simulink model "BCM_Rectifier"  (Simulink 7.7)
settings: Solver=ode45  StartTime=0.0  StopTime=5  RelTol=3e-14
libraries: fl_lib x5, nesl_utility x4, Memristor_lib x1

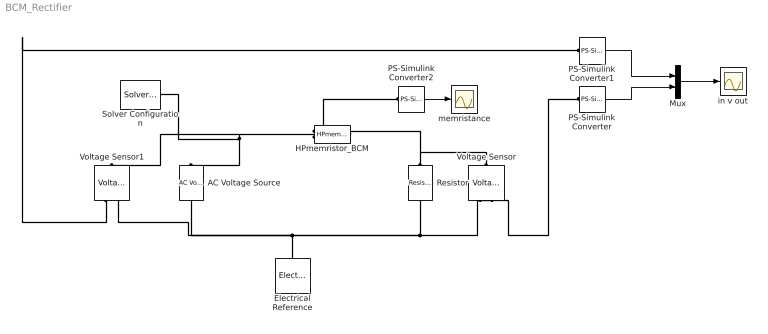
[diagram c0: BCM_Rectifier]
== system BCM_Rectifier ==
  AC Voltage Source : fl_lib/Electrical/Electrical Sources/AC Voltage Source  SystemSampleTime=-1  amp=1 V  shift=0 rad  omega=1 Hz  i_Log=off  v_Log=off  LocalVarNames=|i|v  LocalVarDescs=|i|v  LocalVarLogging=[0 0]
  Electrical Reference : fl_lib/Electrical/Electrical Elements/Electrical Reference  SystemSampleTime=-1  i_Log=off  LocalVarNames=|i  LocalVarDescs=|i  LocalVarLogging=0
  HPmemristor_BCM : Memristor_lib/HPmemristor_BCM  SystemSampleTime=-1  G_off=6e-5 1/Ohm  G_on=0.5 1/Ohm  N=1 1/Ohm  u_v=1e-10 m^2/s/V  D=1e-8 m  x0=0 Ohm  t0=1.1212e-005 s  i0=1 A  VT1=.9 V  VT0=0 V  i_Log=off  v_Log=off  x_Log=off  F_Log=off  W_Log=off  LocalVarNames=|i|v|x|F|W  LocalVarDescs=|i|v|x|F|W  LocalVarLogging=[0 0 0 0 0]
  Mux : Mux  Inputs=2
  PS-Simulink Converter : nesl_utility/PS-Simulink Converter  SystemSampleTime=-1  PhysicalDomain=network_engine_domain  LeftPortType=input  RightPortType=output  SubClassName=ps_output  Unit=1  AffineConversion=off
  PS-Simulink Converter1 : nesl_utility/PS-Simulink Converter  SystemSampleTime=-1  PhysicalDomain=network_engine_domain  LeftPortType=input  RightPortType=output  SubClassName=ps_output  Unit=1  AffineConversion=off
  PS-Simulink Converter2 : nesl_utility/PS-Simulink Converter  SystemSampleTime=-1  PhysicalDomain=network_engine_domain  LeftPortType=input  RightPortType=output  SubClassName=ps_output  Unit=1  AffineConversion=off
  Resistor : fl_lib/Electrical/Electrical Elements/Resistor  SystemSampleTime=-1  R=50 Ohm  i_Log=off  v_Log=off  LocalVarNames=|i|v  LocalVarDescs=|i|v  LocalVarLogging=[0 0]
  Solver Configuration : nesl_utility/Solver Configuration  SystemSampleTime=-1  PhysicalDomain=network_engine_domain  LeftPortType=input  RightPortType=generic  SubClassName=solver  Accelerate=off  Profile=off  ResidualTolerance=1e-9  MaxNonlinIter=3  MaxModeIter=2  DoFixedCost=off  UseLocalSampling=off  DoDC=off  LinearAlgebra=Sparse  LocalSolverSampleTime=.001  LocalSolverChoice=NE_BACKWARD_EULER_ADVANCER  UseLocalSolver=off
  Voltage Sensor : fl_lib/Electrical/Electrical Sensors/Voltage Sensor  SystemSampleTime=-1  i1_Log=off  v1_Log=off  LocalVarNames=|i1|v1  LocalVarDescs=|i1|v1  LocalVarLogging=[0 0]
  Voltage Sensor1 : fl_lib/Electrical/Electrical Sensors/Voltage Sensor  SystemSampleTime=-1  i1_Log=off  v1_Log=off  LocalVarNames=|i1|v1  LocalVarDescs=|i1|v1  LocalVarLogging=[0 0]
  in v out : Scope
  memristance : Scope
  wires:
  PS-Simulink Converter2/1 -> memristance/1
  Mux/1 -> in v out/1
  PS-Simulink Converter1/1 -> Mux/1
  PS-Simulink Converter/1 -> Mux/2
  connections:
  Voltage Sensor/LConn1 -- HPmemristor_BCM/RConn1 -- Resistor/LConn1
  Electrical Reference/LConn1 -- AC Voltage Source/RConn1 -- Voltage Sensor1/RConn2 -- Voltage Sensor/RConn2 -- Resistor/RConn1
  HPmemristor_BCM/LConn1 -- AC Voltage Source/LConn1 -- Solver Configuration/RConn1 -- Voltage Sensor1/LConn1
  PS-Simulink Converter/LConn1 -- Voltage Sensor/RConn1
  Voltage Sensor1/RConn1 -- PS-Simulink Converter1/LConn1
  HPmemristor_BCM/RConn2 -- PS-Simulink Converter2/LConn1
